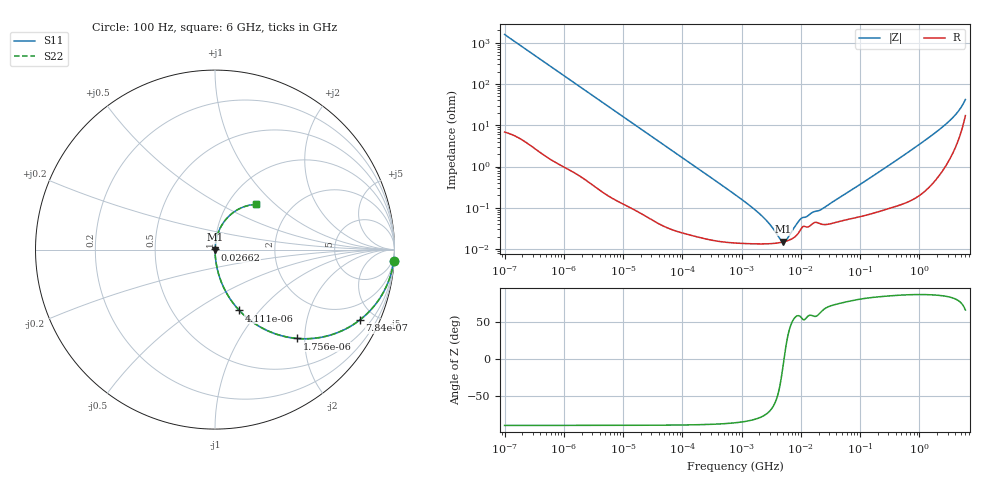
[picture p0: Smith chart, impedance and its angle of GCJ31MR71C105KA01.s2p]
!Murata Part Number: GCJ31MR71C105KA01
!These Parameters are Measured in Series Mode Connection
!Data Generated on Mar 13, 2026
!  o--ll--o
!Port1  Port2
!  o------o
!Operation Temp=25[degC], DC Bias Voltage=0[V]
!Freq. Start=100[Hz] Stop=6[GHz] 401[Steps]
# Hz S RI R 50
!Freq.(Hz) S11(Real) S11(Imag) S21(Real) S21(Imag) S12(Real) S12(Imag) S22(Real) S22(Imag)
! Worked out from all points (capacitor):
!   401 points, 100 Hz to 6 GHz, reference 50 ohm
!   read as one part in series: C = 997 nF near 109 Hz
!   lowest |Z| = 15 mohm at 5.079 MHz (marker M1)
!   series resonance near 5.217 MHz, so ESL is about 930 pH
!   S11 on the Smith chart (normalised r, x): 100 Hz: 1, -32; 784 Hz: 1.02, -4.10; 1.756 kHz: 1.01, -1.84; 4.111 kHz: 1.01, -0.79; 26.62 MHz: 1.00, +0.00; 6 GHz: 1.34, +0.77
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100  0.9958 -0.0624  0.00419 0.0624  0.00419 0.0624  0.9958 -0.0624
366  0.9493 -0.2167  0.0507 0.2167  0.0507 0.2167  0.9493 -0.2167
784  0.8061 -0.3925  0.1939 0.3925  0.1939 0.3925  0.8061 -0.3925
1756  0.4576 -0.4948  0.5424 0.4948  0.5424 0.4948  0.4576 -0.4948
2008  0.3928 -0.485  0.6072 0.485  0.6072 0.485  0.3928 -0.485
4111  0.1358 -0.3392  0.8642 0.3392  0.8642 0.3392  0.1358 -0.3392
11514  0.0206 -0.138  0.9794 0.138  0.9794 0.138  0.0206 -0.138
40335  0.00204 -0.0404  0.998 0.0404  0.998 0.0404  0.00204 -0.0404
774597  0.000144 -0.00209  0.9999 0.00209  0.9999 0.00209  0.000144 -0.00209
2268635  0.000134 -0.000597  0.9999 0.000597  0.9999 0.000597  0.000134 -0.000597
3103719  0.000135 -0.000349  0.9999 0.000349  0.9999 0.000349  0.000135 -0.000349
4440638  0.000143 -0.000105  0.9999 0.000105  0.9999 0.000105  0.000143 -0.000105
5079039  0.000149 -1.72e-05  0.9999 1.72e-05  0.9999 1.72e-05  0.000149 -1.72e-05
5809218  0.000157 7.06e-05  0.9998 -7.06e-05  0.9998 -7.06e-05  0.000157 7.06e-05
9941735  0.000297 0.00045  0.9997 -0.00045  0.9997 -0.00045  0.000297 0.00045
1.555665e7  0.000404 0.000654  0.9996 -0.000654  0.9996 -0.000654  0.000404 0.000654
2.662322e7  0.000394 0.00101  0.9996 -0.00101  0.9996 -0.00101  0.000394 0.00101
3.124326e8  0.00108 0.0108  0.9989 -0.0108  0.9989 -0.0108  0.00108 0.0108
1.251881e9  0.00439 0.043  0.9956 -0.043  0.9956 -0.043  0.00439 0.043
3.065283e9  0.0261 0.1141  0.9739 -0.1141  0.9739 -0.1141  0.0261 0.1141
4.586474e9  0.0823 0.1908  0.9177 -0.1908  0.9177 -0.1908  0.0823 0.1908
6e9  0.2299 0.2528  0.7701 -0.2528  0.7701 -0.2528  0.2299 0.2528
